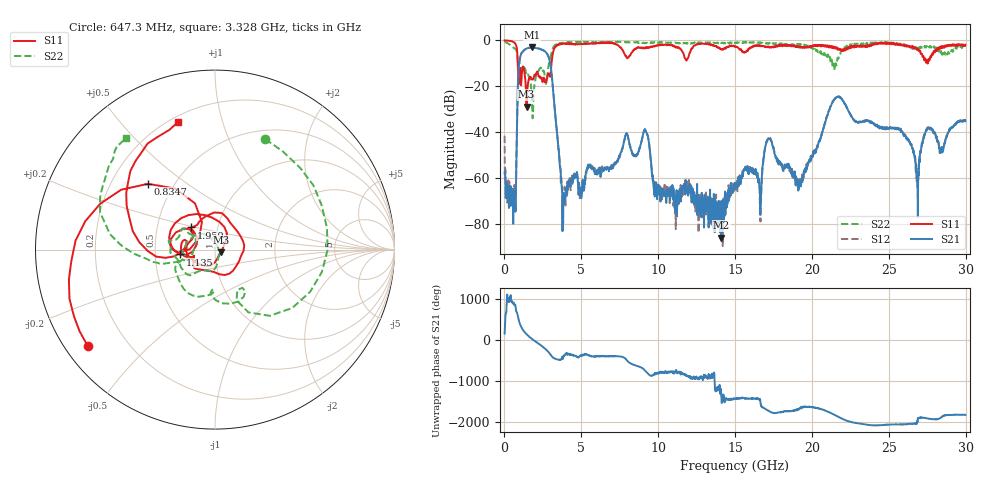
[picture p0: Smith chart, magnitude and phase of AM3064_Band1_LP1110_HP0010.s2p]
# Hz S DB R 50.0
!freq dBS11 angS11 dBS21 angS21 dBS12 angS12 dBS22 angS22
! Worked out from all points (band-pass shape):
!   1600 points, 10 MHz to 29.98 GHz, reference 50 ohm
!   highest |S21| = -3.07 dB at 1.791 GHz (marker M1); lowest = -85.9 dB at 14.11 GHz (marker M2)
!   |S21| within 3 dB of the highest: 1.077 GHz to 2.796 GHz (1.719 GHz wide, 88.8 % of centre)
!   lowest |S11| = -28.8 dB at 1.435 GHz (marker M3), VSWR 1.08, Z = 53.4 - j1.51 ohm
!   |S11| at or under -10 dB: 866.1 MHz to 3.06 GHz (2.194 GHz wide, 112 % of centre); 27.52423 GHz to 27.53536 GHz (11.13 MHz wide, 0.0404 % of centre)
!   |S22| runs from -33.9 to -0.4 dB; largest |S21 - S12| = 0.012
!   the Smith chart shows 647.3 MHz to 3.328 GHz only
!   S11 on the Smith chart (normalised r, x): 647.3 MHz: 0.07, -0.33; 834.7 MHz: 0.36, +0.36; 1.135 GHz: 0.67, -0.04; 1.959 GHz: 0.75, +0.19; 3.328 GHz: 0.23, +0.73
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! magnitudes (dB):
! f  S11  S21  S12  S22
! 10 MHz  0.0  -58.0  -41.6  -0.4
! 647.3 MHz  -1.0  -66.7  -63.0  -3.4
! 834.7 MHz  -5.6  -30.6  -30.6  -6.4
! 1.135 GHz  -14.1  -5.3  -5.3  -12.3
! 1.435 GHz  -28.8  -3.5  -3.5  -15.2
! 1.791 GHz  -16.8  -3.1  -3.1  -27.3
! 1.959 GHz  -14.9  -3.2  -3.2  -18.8
! 2.878 GHz  -14.4  -7.3  -7.3  -10.5
! 3.328 GHz  -2.6  -34.0  -34.1  -2.0
! 3.834 GHz  -1.4  -69.7  -71.6  -1.1
! 5.015 GHz  -1.4  -64.0  -68.4  -0.7
! 9.157 GHz  -3.3  -39.0  -38.9  -1.1
! 10 GHz  -2.2  -64.7  -64.4  -0.9
! 14.11 GHz  -3.9  -85.9  -72.8  -1.1
! 15 GHz  -2.6  -63.3  -62.4  -1.2
! 16.62 GHz  -2.1  -67.5  -73.3  -0.9
! 17.2 GHz  -2.7  -43.0  -42.6  -1.1
! 19.99 GHz  -2.8  -50.8  -51.1  -3.1
! 21.64 GHz  -3.2  -24.7  -24.7  -8.6
! 25 GHz  -1.0  -38.4  -38.0  -1.1
! 26.85 GHz  -4.3  -62.4  -61.5  -2.8
! 29.98 GHz  -1.9  -35.2  -35.0  -2.8
